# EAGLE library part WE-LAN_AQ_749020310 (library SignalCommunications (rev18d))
WE-LAN AQ 10/100 Base-T SMD Transformer 1 Port Characteristics 100 % machine production High performance return loss and crosstalk Improved solderability through half vias Reduced height (4 mm) Compatible to standard products Applications Compatible to industrial ethernet systems like EtherCAT or Profinet IoT applications Hubs, routers, switches, IPcameras Company networks Details see: http://katalog.we-online.de/en/pbs/WE-LANAQ Created by Yingchun Shan 2017 (C) Wurth Elektronik
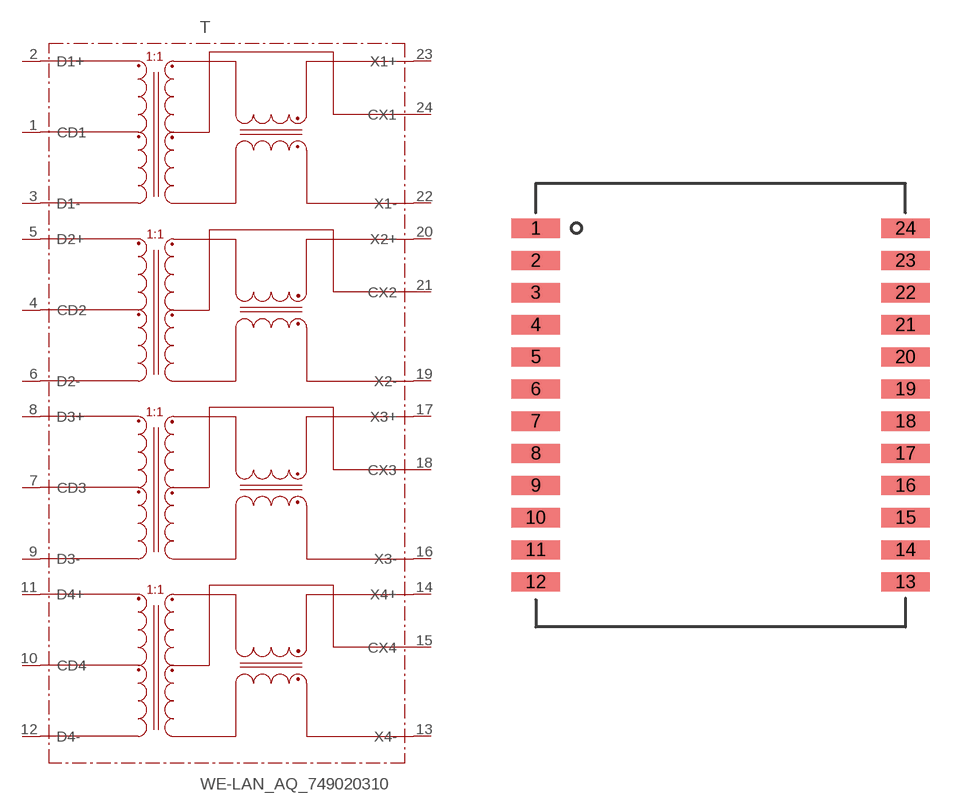
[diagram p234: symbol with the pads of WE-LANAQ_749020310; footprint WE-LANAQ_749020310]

Designator prefix T

## WE-LAN_AQ_749020310  [WE-LANAQ_749020310]
1  CD1
2  D1+
3  D1-
4  CD2
5  D2+
6  D2-
7  CD3
8  D3+
9  D3-
10  CD4
11  D4+
12  D4-
13  X4-
14  X4+
15  CX4
16  X3-
17  X3+
18  CX3
19  X2-
20  X2+
21  CX2
22  X1-
23  X1+
24  CX1

## Footprint WE-LANAQ_749020310 (pad centres in mm)
smd 1.9 x 0.76: 1 -7.305,6.985; 2 -7.305,5.715; 3 -7.305,4.445; 4 -7.305,3.175; 5 -7.305,1.905; 6 -7.305,0.635; 7 -7.305,-0.635; 8 -7.305,-1.905; 9 -7.305,-3.175; 10 -7.305,-4.445; 11 -7.305,-5.715; 12 -7.305,-6.985; 13 7.305,-6.985; 14 7.305,-5.715; 15 7.305,-4.445; 16 7.305,-3.175; 17 7.305,-1.905; 18 7.305,-0.635; 19 7.305,0.635; 20 7.305,1.905; 21 7.305,3.175; 22 7.305,4.445; 23 7.305,5.715; 24 7.305,6.985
